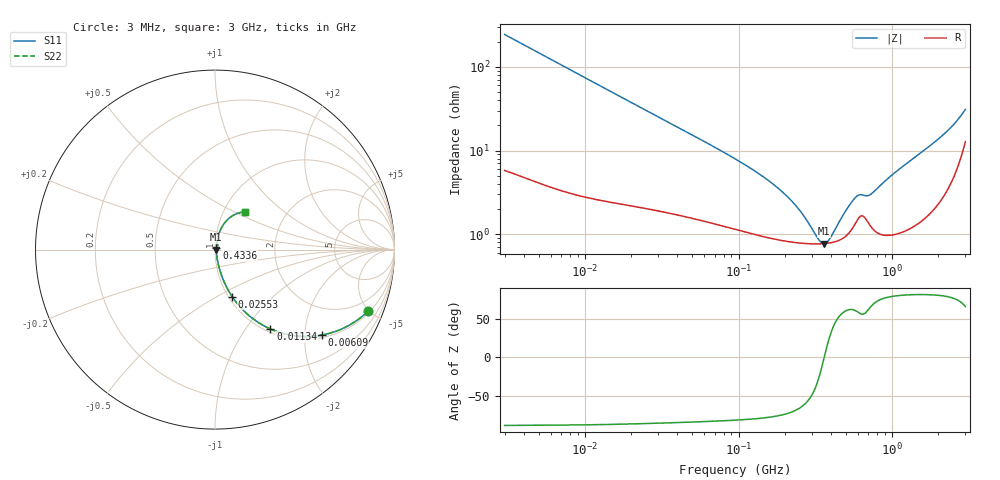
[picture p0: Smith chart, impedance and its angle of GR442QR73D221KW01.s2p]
!Murata Part Number: GR442QR73D221KW01
!These Parameters are Measured in Series Mode Connection
!Data Generated on Mar 13, 2026
!  o--ll--o
!Port1  Port2
!  o------o
!Operation Temp=25[degC], DC Bias Voltage=0[V]
!Freq. Start=3[MHz] Stop=3[GHz] 401[Steps]
# Hz S RI R 50
!Freq.(Hz) S11(Real) S11(Imag) S21(Real) S21(Imag) S12(Real) S12(Imag) S22(Real) S22(Imag)
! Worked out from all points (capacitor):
!   401 points, 3 MHz to 3 GHz, reference 50 ohm
!   read as one part in series: C = 216 pF near 3.105 MHz
!   lowest |Z| = 771 mohm at 358.6 MHz (marker M1)
!   series resonance near 361.5 MHz, so ESL is about 900 pH
!   S11 on the Smith chart (normalised r, x): 3 MHz: 1.12, -4.88; 6.09 MHz: 1.07, -2.43; 11.34 MHz: 1.05, -1.31; 25.53 MHz: 1.04, -0.59; 433.6 MHz: 1.02, +0.02; 3 GHz: 1.26, +0.57
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3000000  0.8506 -0.3448  0.1494 0.3448  0.1494 0.3448  0.8506 -0.3448
6090056  0.5934 -0.4766  0.4066 0.4766  0.4066 0.4766  0.5934 -0.4766
9541601  0.3819 -0.468  0.6181 0.468  0.6181 0.468  0.3819 -0.468
1.134021e7  0.3085 -0.4422  0.6915 0.4422  0.6915 0.4422  0.3085 -0.4422
1.687024e7  0.1771 -0.3567  0.8229 0.3567  0.8229 0.3567  0.1771 -0.3567
2.553414e7  0.0954 -0.2618  0.9046 0.2618  0.9046 0.2618  0.0954 -0.2618
3.034738e7  0.0739 -0.2266  0.9261 0.2266  0.9261 0.2266  0.0739 -0.2266
9.486833e7  0.0173 -0.0767  0.9827 0.0767  0.9827 0.0767  0.0173 -0.0767
1.43589e8  0.0115 -0.0472  0.9885 0.0472  0.9885 0.0472  0.0115 -0.0472
1.959392e8  0.00914 -0.0296  0.9909 0.0296  0.9909 0.0296  0.00914 -0.0296
2.452569e8  0.00813 -0.0183  0.9919 0.0183  0.9919 0.0183  0.00813 -0.0183
3.017319e8  0.00766 -0.00847  0.9923 0.00847  0.9923 0.00847  0.00766 -0.00847
3.346734e8  0.0076 -0.00363  0.9924 0.00363  0.9924 0.00363  0.0076 -0.00363
3.586091e8  0.00764 -0.000384  0.9924 0.000384  0.9924 0.000384  0.00764 -0.000384
3.842565e8  0.00775 0.0029  0.9922 -0.0029  0.9922 -0.0029  0.00775 0.0029
4.336319e8  0.00821 0.00884  0.9918 -0.00884  0.9918 -0.00884  0.00821 0.00884
5.153725e8  0.0102 0.0179  0.9898 -0.0179  0.9898 -0.0179  0.0102 0.0179
5.815958e8  0.0142 0.0235  0.9858 -0.0235  0.9858 -0.0235  0.0142 0.0235
7.155191e8  0.0134 0.0258  0.9866 -0.0258  0.9866 -0.0258  0.0134 0.0258
9.596685e8  0.0117 0.0459  0.9883 -0.0459  0.9883 -0.0459  0.0117 0.0459
2.123837e9  0.0461 0.1382  0.9539 -0.1382  0.9539 -0.1382  0.0461 0.1382
3e9  0.1658 0.2095  0.8342 -0.2095  0.8342 -0.2095  0.1658 0.2095
